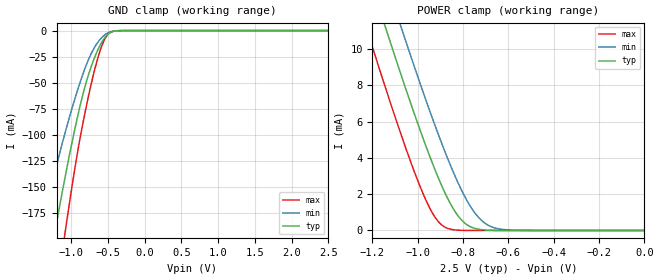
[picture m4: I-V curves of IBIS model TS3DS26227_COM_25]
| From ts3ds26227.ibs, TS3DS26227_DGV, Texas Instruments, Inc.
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[Model]   TS3DS26227_COM_25
Model_type  Terminator
| variable   typ   min   max
C_comp   8.68pF   6.51pF   10.59pF
| C_tri-state   8.68pF   6.51pF   10.59pF
[Temperature Range]   40   100   -40
| Ambient temperature   25   85   -40
[Voltage range]   2.5   2.3   2.7
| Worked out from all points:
|   GND clamp passes 1 mA (typ) near -0.44 V on its own axis
|   POWER clamp passes 1 mA (typ) near -0.83 V on its own axis
[GND Clamp]
| TS3DS26227_COM_25
|   Voltage   I(typ)   I(min)   I(max)
-2.5V     -772.7mA   -579mA     -951.3mA
-1.425V   -275.4mA   -195.1mA   -366.6mA
-1.395V   -262.8mA   -185.9mA   -350.9mA
-1.235V   -197.9mA   -138.9mA   -268.5mA
-1.21V    -188.1mA   -131.8mA   -255.9mA
-1.075V   -137.3mA   -95.7mA    -189.3mA
-915mV    -82.89mA   -57.31mA   -116.9mA
-775mV    -44.52mA   -29.44mA   -65.98mA
-625mV    -16.51mA   -9.995mA   -23.24mA
-510mV    -4.087mA   -2.512mA   -4.475mA
-330mV    -66.36uA   -63.28uA   -26.45uA
2.5V      6.067nA    10.91nA    2.751nA
[POWER Clamp]
| TS3DS26227_COM_25
|   Voltage   I(typ)   I(min)   I(max)
-2.5V     67.33mA    69.82mA    64.3mA
-1.245V   15.22mA    17.89mA    11.89mA
-1.21V    13.84mA    16.5mA     10.5mA
-1.15V    11.49mA    14.15mA    8.16mA
-1.125V   10.53mA    13.19mA    7.204mA
-1.075V   8.634mA    11.28mA    5.339mA
-975mV    5.025mA    7.58mA     1.983mA
-910mV    2.924mA    5.324mA    501.7uA
-810mV    618.6uA    2.304mA    9.384uA
-710mV    34.34uA    462.1uA    109nA
-600mV    896.2nA    27.97uA    3.744nA
-31.15fV  6.067nA    10.26nA    2.824nA
